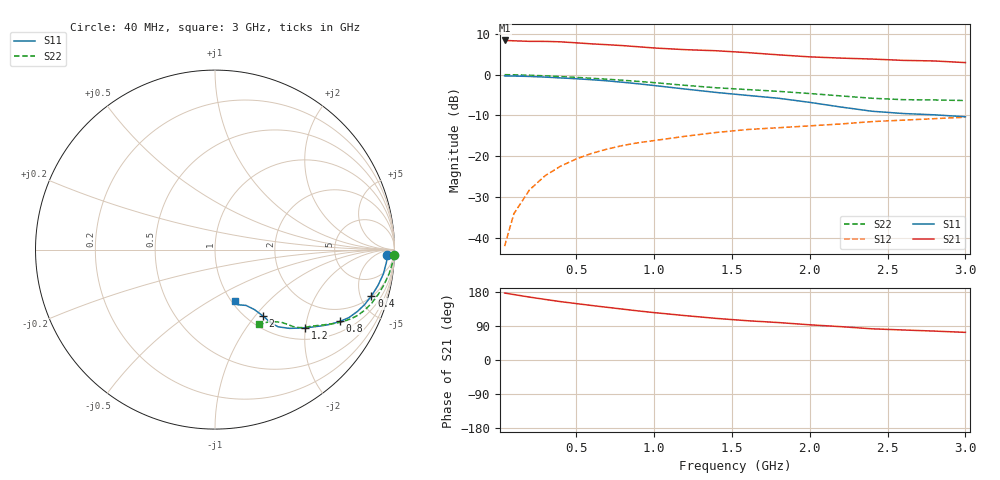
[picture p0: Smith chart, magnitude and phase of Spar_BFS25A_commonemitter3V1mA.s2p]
! Filename:  BFS25AI.S2P  Version:  4.0
! NXP part #: BFS25A  Date: Jun 1994
! Bias condition: Vce=3V, Ic=1mA
#  MHz  S  MA  R  50
! Freq  S11  S21  S12  S22  !GUM [dB]
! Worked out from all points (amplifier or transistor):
!   21 points, 40 MHz to 3 GHz, reference 50 ohm
!   highest |S21| = 8.3 dB at 40 MHz (marker M1)
!   |S21| within 3 dB of that: start of sweep to 1.611 GHz
!   unconditionally stable (mu >= 1): 2.075 GHz to end of sweep
!   at 300 MHz: K = 0.23, MSG = 16.4 dB, |S12| = -24.7 dB
!   at 1 GHz: K = 0.58, MSG = 11.3 dB, |S12| = -16.1 dB
!   at 3 GHz: K = 1.09, MAG = 4.8 dB, |S12| = -10.4 dB
!   lowest NFmin = 1.90 dB at 500 MHz
!   S11 on the Smith chart (normalised r, x): 40 MHz: 32, -24; 400 MHz: 2.09, -6.21; 800 MHz: 1.41, -3.18; 1.2 GHz: 1.27, -1.99; 2 GHz: 1.18, -1.10; 3 GHz: 1.04, -0.65
40  0.961 -1.7  2.608 176.7  0.008 89.6  0.996 -1.6
100  0.958 -4.1  2.582 172.7  0.02 85.5  0.993 -3.9
200  0.948 -8.2  2.544 166.0  0.039 81.5  0.98 -7.7
300  0.93 -12.4  2.541 159.9  0.058 78.3  0.963 -11.5
400  0.909 -16.5  2.509 154.0  0.076 75.5  0.944 -15.2
500  0.888 -20.2  2.441 148.9  0.093 72.8  0.923 -18.8
600  0.864 -23.6  2.369 143.8  0.109 70.5  0.9 -22.0
700  0.837 -26.9  2.314 139.0  0.123 68.5  0.876 -24.7
800  0.804 -29.8  2.255 134.2  0.136 66.6  0.851 -26.9
900  0.77 -32.6  2.183 129.4  0.147 64.5  0.824 -28.9
1000  0.734 -35.3  2.111 125.1  0.156 62.6  0.797 -30.8
1200  0.665 -41.0  2.013 117.1  0.176 59.0  0.738 -34.6
1400  0.604 -46.6  1.952 109.8  0.196 56.6  0.689 -38.2
1600  0.556 -50.7  1.853 103.6  0.213 54.5  0.655 -41.6
1800  0.513 -52.7  1.74 98.8  0.224 53.7  0.623 -44.1
2000  0.457 -54.1  1.644 92.9  0.236 52.4  0.586 -45.6
2200  0.401 -56.6  1.587 88.0  0.249 51.5  0.548 -47.6
2400  0.356 -60.9  1.546 82.3  0.266 49.9  0.513 -51.4
2600  0.334 -67.0  1.489 79.2  0.277 48.6  0.493 -55.6
2800  0.322 -69.6  1.465 76.3  0.289 49.1  0.489 -58.3
3000  0.305 -68.5  1.399 72.9  0.301 48.6  0.481 -59.4
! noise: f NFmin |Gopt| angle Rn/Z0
500  1.9  0.839  3  2.4
1000  2  0.775  9  2.4
2000  2.3  0.804  26  1.6
